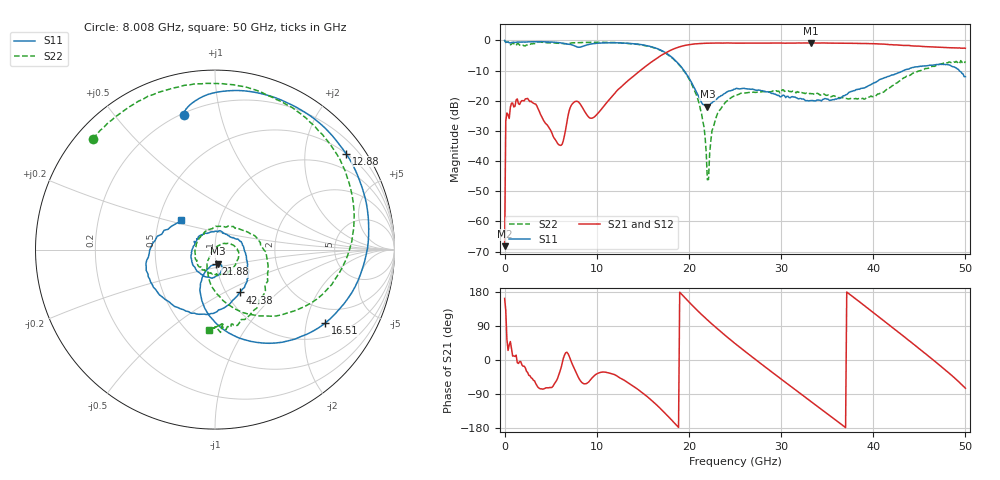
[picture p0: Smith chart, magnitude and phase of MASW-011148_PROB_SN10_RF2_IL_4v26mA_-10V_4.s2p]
!Keysight Technologies,N5247A,US51170177,A.10.64.09
!Date: Saturday, May 29, 2021 13:16:39
!Correction: S11(Full 2 Port(1,2))
!S21(Full 2 Port(1,2))
!S12(Full 2 Port(1,2))
!S22(Full 2 Port(1,2))
!S2P File: Measurements: S11, S21, S12, S22:
# Hz S  dB  R 50
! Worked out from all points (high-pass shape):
!   401 points, 10 MHz to 50 GHz, reference 50 ohm
!   highest |S21| = -0.83 dB at 33.25 GHz (marker M1); lowest = -68.2 dB at 10 MHz (marker M2)
!   |S21| within 3 dB of the highest: 17.65 GHz to end of sweep
!   lowest |S11| = -21.9 dB at 22.01 GHz (marker M3), VSWR 1.17, Z = 50.8 - j8.07 ohm
!   |S11| at or under -10 dB: 19.47 GHz to 43.27 GHz (23.8 GHz wide, 75.9 % of centre); 49.33 GHz to end of sweep
!   |S22| runs from -46.2 to 0.0 dB; largest |S21 - S12| = 0.03
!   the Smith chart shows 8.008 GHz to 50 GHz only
!   S11 on the Smith chart (normalised r, x): 8.008 GHz: 0.21, +0.77; 12.88 GHz: 0.51, +2.98; 16.51 GHz: 1.43, -2.58; 21.88 GHz: 1.00, -0.16; 42.38 GHz: 1.16, -0.60; 50 GHz: 0.65, +0.23
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1e7  -0.01 -1.8  -68.18 162.5  -71.73 154.2  -0.02 -0.9
3.84925e8  -0.60 -51.5  -24.64 25.2  -24.62 25.2  -0.43 -25.4
1.25975e9  -0.66 -121.4  -19.72 12.8  -19.71 12.9  -1.70 -67.4
2.384525e9  -0.51 -163.8  -19.31 -29.4  -19.29 -29.3  -1.52 -107.0
6.0088e9  -0.77 126.8  -34.73 -30.6  -34.67 -30.7  -0.98 167.1
8.0084e9  -2.27 103.1  -20.35 -45.6  -20.32 -45.6  -0.75 137.8
8.383325e9  -2.07 102.4  -21.91 -59.1  -21.89 -59.1  -0.72 132.3
1.288242e10  -0.87 36.2  -14.79 -52.1  -14.76 -51.9  -0.91 63.7
1.65067e10  -2.64 -33.8  -5.94 -118.7  -5.89 -118.6  -2.76 -5.2
1.675665e10  -2.96 -39.6  -5.43 -124.4  -5.38 -124.4  -3.05 -10.8
2.038092e10  -14.47 -113.4  -1.25 143.8  -1.22 143.7  -15.00 -99.9
2.188062e10  -21.77 -85.6  -0.93 108.5  -0.92 108.4  -37.06 -154.4
2.20056e10  -21.91 -79.4  -0.93 105.7  -0.91 105.7  -46.16 -179.2
2.5005e10  -16.13 -93.7  -0.90 43.6  -0.80 43.5  -18.24 2.7
2.85043e10  -17.02 -160.3  -0.89 -22.5  -0.85 -22.8  -16.88 -44.3
3.325335e10  -19.95 102.9  -0.83 -109.5  -0.87 -109.9  -17.65 -110.9
3.337832e10  -19.93 100.5  -0.84 -111.9  -0.86 -112.2  -17.65 -114.7
3.737752e10  -17.20 25.1  -0.94 174.6  -0.94 174.8  -19.41 166.9
4.175165e10  -11.84 -47.5  -1.39 91.6  -1.25 92.2  -15.74 46.5
4.237652e10  -11.14 -59.4  -1.48 79.9  -1.33 80.3  -14.40 34.2
4.625075e10  -8.22 -128.7  -2.14 5.2  -2.07 4.5  -8.71 -41.3
5e10  -12.01 139.3  -2.61 -74.5  -2.68 -75.3  -6.94 -94.0
